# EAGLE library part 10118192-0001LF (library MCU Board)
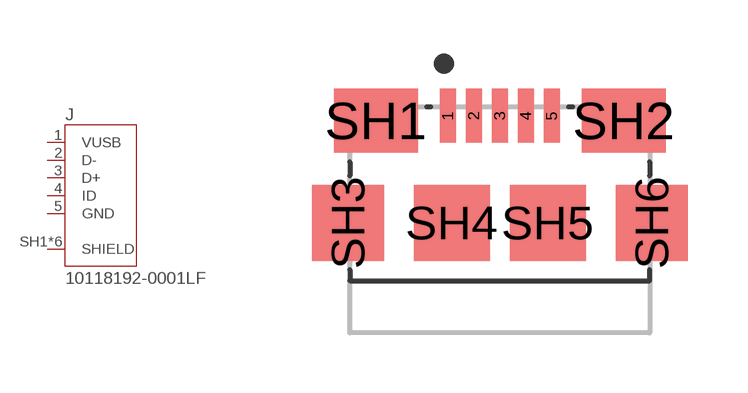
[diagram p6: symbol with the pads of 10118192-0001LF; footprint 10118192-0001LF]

Designator prefix J

## 10118192-0001LF  [10118192-0001LF]
1  VUSB  pas
2  D-  pas
3  D+  pas
4  ID  pas
5  GND  pas
SH1  SHIELD  pas
SH2  SHIELD  pas
SH3  SHIELD  pas
SH4  SHIELD  pas
SH5  SHIELD  pas
SH6  SHIELD  pas

## Footprint 10118192-0001LF (pad centres in mm)
smd 0.4 x 1.35: 1 -1.3,2.54; 2 -0.65,2.54; 3 0,2.54; 4 0.65,2.54; 5 1.3,2.54
smd 2.1 x 1.6: SH1 -3.1,2.415; SH2 3.1,2.415
smd 1.8 x 1.9: SH3 -3.8,-0.135; SH6 3.8,-0.135
smd 1.9 x 1.9: SH4 -1.2,-0.135; SH5 1.2,-0.135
